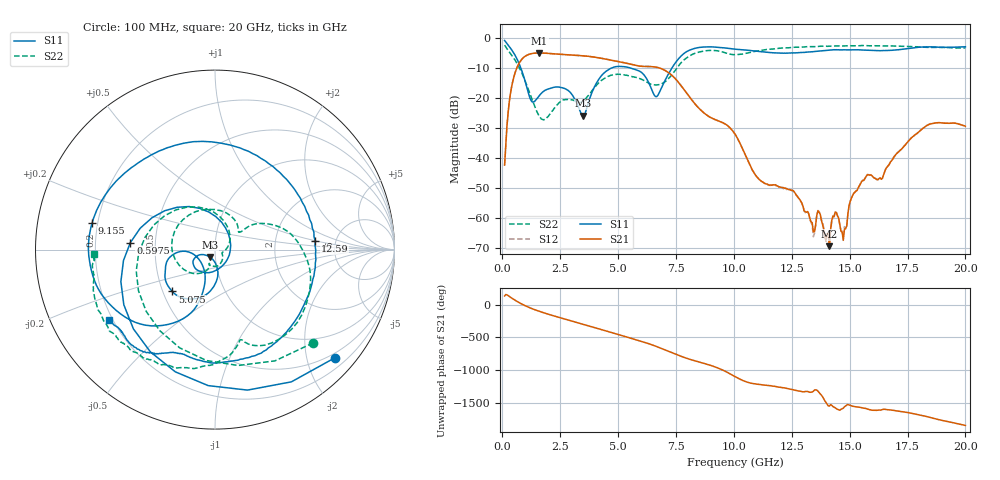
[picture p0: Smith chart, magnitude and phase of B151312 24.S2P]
!  2-Port S-parameters saved by WinCal
! VAR MeasName=S-Parameters (CALIBRATED_DATA) read from VNA (N5244A)
! VAR MeasDate=12/8/2015 5:45:15 PM
! VAR NAME=B151312 24
! VAR FILENAME=B151312 24.S2P
! VAR DATE=12/8/2015 5:45:15 PM
! VAR PHYS_PORTS=1,2
# Hz S DB R 50
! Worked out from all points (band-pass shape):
!   401 points, 100 MHz to 20 GHz, reference 50 ohm
!   highest |S21| = -5.08 dB at 1.593 GHz (marker M1); lowest = -69.4 dB at 14.13 GHz (marker M2)
!   |S21| within 3 dB of the highest: 759.1 MHz to 5.116 GHz (4.357 GHz wide, 148 % of centre)
!   lowest |S11| = -26.0 dB at 3.483 GHz (marker M3), VSWR 1.11, Z = 47 - j3.87 ohm
!   |S11| at or under -10 dB: 796.5 MHz to 4.744 GHz (3.947 GHz wide, 142 % of centre); 5.502 GHz to 7.333 GHz (1.831 GHz wide, 28.5 % of centre)
!   |S22| runs from -27.3 to -2.4 dB; largest |S21 - S12| = 0.0013
!   S11 on the Smith chart (normalised r, x): 100 MHz: 0.40, -2.56; 597.5 MHz: 0.36, +0.04; 5.075 GHz: 0.56, -0.29; 9.155 GHz: 0.18, +0.10; 12.59 GHz: 3.48, +0.48; 20 GHz: 0.19, -0.29
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1e8  -0.91 -41.9  -42.41 134.9  -42.41 136.5  -2.45 -43.5
3.4875e8  -3.43 -122.3  -18.74 116.5  -18.74 116.5  -5.25 -124.3
5.975e8  -6.50 175.3  -10.66 59.7  -10.66 59.6  -8.05 170.1
1.04525e9  -16.10 76.2  -5.88 -23.8  -5.89 -23.8  -15.57 72.4
1.5925e9  -19.34 -78.1  -5.08 -99.6  -5.08 -99.6  -26.11 -12.0
2.3885e9  -16.38 -135.5  -5.45 172.8  -5.45 172.7  -22.22 -63.1
3.43325e9  -25.58 -136.8  -5.99 67.1  -5.99 67.1  -21.39 -111.8
3.483e9  -25.99 -125.2  -6.02 62.1  -6.02 62.0  -21.11 -110.2
4.1795e9  -13.69 -92.1  -6.71 -9.9  -6.70 -9.9  -14.89 -132.4
5.075e9  -9.54 -135.6  -8.00 -102.5  -8.00 -102.4  -12.16 146.2
5.871e9  -10.94 -163.7  -9.39 173.8  -9.37 173.7  -13.39 72.7
6.7665e9  -18.49 -123.1  -10.03 65.6  -10.03 65.6  -15.61 35.6
7.91075e9  -4.87 -132.4  -17.89 -94.1  -17.88 -94.4  -7.00 8.6
9.1545e9  -3.10 167.8  -27.12 132.0  -27.14 131.5  -4.25 -54.7
1.005e10  -3.80 131.8  -32.05 -20.3  -32.12 -20.6  -5.64 -74.4
1.109475e10  -4.58 83.9  -47.20 -141.5  -47.26 -140.9  -4.31 -84.8
1.258725e10  -5.03 4.8  -51.07 134.7  -51.19 134.2  -3.17 -108.0
1.338325e10  -4.67 -32.1  -61.52 102.9  -62.35 106.3  -2.99 -117.7
1.41295e10  -4.12 -59.7  -69.38 -113.6  -69.35 -106.0  -2.84 -127.2
1.67165e10  -4.22 -111.0  -42.13 -170.6  -41.93 -170.6  -2.70 -153.0
1.8408e10  -3.02 -131.4  -28.93 78.2  -28.88 78.4  -3.21 -167.0
2e10  -3.01 -146.2  -29.48 -50.0  -29.55 -51.1  -3.42 -178.1
